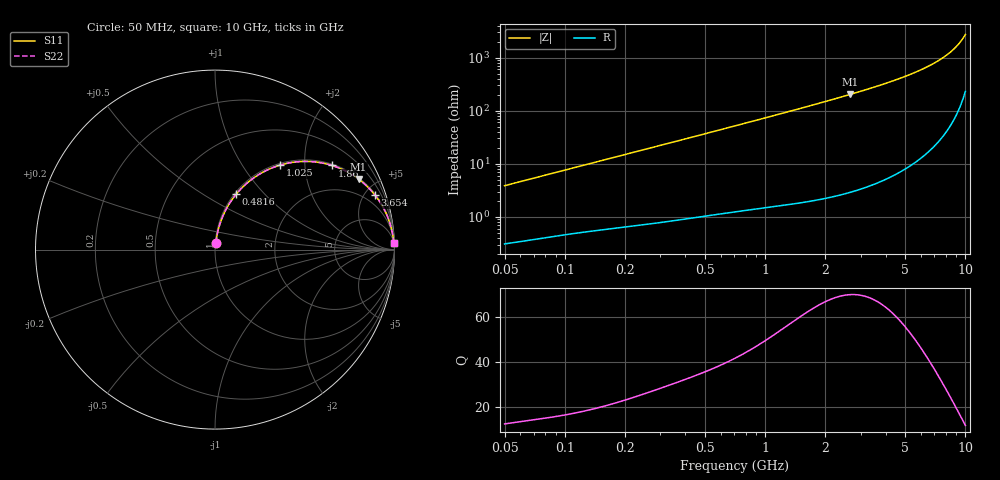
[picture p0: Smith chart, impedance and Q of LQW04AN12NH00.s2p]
!Murata Part Number: LQW04AN12NH00
!These Parameters are Measured in Series Mode Connection
!  o--[Z]--o
!Port1  Port2
!  o-------o
!Freq. Start=50[MHz] Stop=10[GHz], 401[Steps]
# Hz S RI R 50
!Freq.(Hz)	S 11(Real)	S 11(Imag)	S 21(Real)	S 21(Imag)	S 12(Real)	S 12(Imag)	S 22(Real)	S 22(Imag)
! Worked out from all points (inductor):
!   401 points, 50 MHz to 10 GHz, reference 50 ohm
!   read as one part in series: L = 12.2 nH near 51.34 MHz
!   highest Q = 69.8 at 2.659 GHz (marker M1), where L = 12.1 nH
!   S11 on the Smith chart (normalised r, x): 50 MHz: 1.01, +0.08; 481.6 MHz: 1.02, +0.70; 1.025 GHz: 1.03, +1.49; 1.86 GHz: 1.04, +2.75; 3.654 GHz: 1.09, +5.83; 10 GHz: 6, +54
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5e7  0.00455 0.0382  0.9954 -0.0382  0.9954 -0.0382  0.00455 0.0382
1.214486e8  0.0132 0.0895  0.9868 -0.0895  0.9868 -0.0895  0.0132 0.0895
1.930779e8  0.026 0.1386  0.974 -0.1386  0.974 -0.1386  0.026 0.1386
2.949953e8  0.0517 0.2043  0.9483 -0.2043  0.9483 -0.2043  0.0517 0.2043
4.81571e8  0.1173 0.3078  0.8827 -0.3078  0.8827 -0.3078  0.1173 0.3078
7.071068e8  0.2157 0.3994  0.7843 -0.3994  0.7843 -0.3994  0.2157 0.3994
1.024606e9  0.361 0.4704  0.639 -0.4704  0.639 -0.4704  0.361 0.4704
1.335391e9  0.4887 0.4912  0.5113 -0.4912  0.5113 -0.4912  0.4887 0.4912
1.717543e9  0.614 0.479  0.386 -0.479  0.386 -0.479  0.614 0.479
1.859615e9  0.652 0.4687  0.348 -0.4687  0.348 -0.4687  0.652 0.4687
2.659148e9  0.7997 0.3931  0.2003 -0.3931  0.2003 -0.3931  0.7997 0.3931
3.654301e9  0.8911 0.304  0.1089 -0.304  0.1089 -0.304  0.8911 0.304
4.171863e9  0.9186 0.2656  0.0814 -0.2656  0.0814 -0.2656  0.9186 0.2656
4.955797e9  0.9463 0.2166  0.0537 -0.2166  0.0537 -0.2166  0.9463 0.2166
5.733131e9  0.9639 0.1766  0.0361 -0.1766  0.0361 -0.1766  0.9639 0.1766
6.54512e9  0.976 0.1415  0.024 -0.1415  0.024 -0.1415  0.976 0.1415
7.276762e9  0.9833 0.1143  0.0167 -0.1143  0.0167 -0.1143  0.9833 0.1143
7.983737e9  0.9883 0.0911  0.0117 -0.0911  0.0117 -0.0911  0.9883 0.0911
8.644138e9  0.9916 0.0716  0.00838 -0.0716  0.00838 -0.0716  0.9916 0.0716
9.236013e9  0.9937 0.0555  0.00627 -0.0555  0.00627 -0.0555  0.9937 0.0555
9.738562e9  0.995 0.0428  0.00497 -0.0428  0.00497 -0.0428  0.995 0.0428
1e10  0.9956 0.0364  0.00444 -0.0364  0.00444 -0.0364  0.9956 0.0364
